| TEXAS INSTRUMENTS INCORPORATED
| Standard Linear and Logic Group
| IBIS Model of SN74CBTLV3861
| LOW-VOLTAGE 10-BIT FET BUS SWITCH
| This file contains package information for the following:
|  TSSOP 24-pin (PW) package as [Component] CBTLV3861_PW
|  TVSOP 24-pin (DGV) package as [Component] CBTLV3861_DGV
|  SOIC 24-pin (DW) package as [Component] CBTLV3861_DW
|  SOP 24-pin (NS) package as [Component] CBTLV3861_NS
|  SSOP 24-pin (DBQ) package as [Component] CBTLV3861_DBQ
| This device can be powered at the following Vccs:
|  3.3 volt Vcc
|  2.5 volt Vcc
| This file provides unique models under the [Model Selector] for each Vcc.
| For operation at a specific Vcc, select the appropriate model after each
| [Model Selector] keyword.
[IBIS Ver]   3.2
[Comment char]  |_char
[File Name]   sn74cbtlv3861.ibs
[File Rev]   1.0 | x_die
[Date]   May 11, 2009
[Source]   Data created from TI-SPICE simulations at TI-SLL.
[Notes]   The following is an IBIS list for the SN74CBTLV3861.
   Please contact sllibis@ti.com with questions and
   comments concerning SLL IBIS models.
   -FILE REV HISTORY
   -1.0 Release IBIS file on 05/11/09.
   -Power clamp data deleted as there is no power-clamp diode.
[Disclaimer] Property of Texas Instruments Incorporated.  Unauthorized
   reproduction and/or distribution is strictly prohibited.
   This product is protected under copyright law.
   Created  2007, (C) Copyright  2007, Texas Instruments
   Incorporated, All Rights Reserved
   UNLESS THERE IS A SIGNED, WRITTEN AGREEMENT TO THE
   CONTRARY, TEXAS INSTRUMENTS (TI) IS PROVIDING THE IBIS
   MODELS  AND WITHOUT ANY WARRANTY, EXPRESSED OR
   IMPLIED.  TI assumes no liability for:
   1) the accuracy of the IBIS models provided to your
   company;
   2) the proper functioning of these IBIS Models in your
   design or for any resulting applications; or
   3) infringement of patents, copyrights or intellectual
   property rights resulting from your use of these IBIS
   models.
   TI provides IBIS Models as a service to our customers.
   You and your company shall not distribute, sell or give
   these models to anyone else without prior written
   permission from TI.
   TI reserves the right to make changes to our products or
   to discontinue any semiconductor product or service
   without notice, and advises our customers to obtain the
   latest version of relevant information to verify, before
   placing orders, that the information being relied on is
   current.
   Please be aware that your receipt and use of the IBIS
   information provided shall serve as acceptance of these
   terms and conditions.  If you do not accept these terms,
   you should return or destroy the IBIS models and any
   other accompanying information immediately.
| Component SN74CBTLV3861_PW 24-PIN TSSOP
[Component]   SN74CBTLV3861_PW
[Manufacturer]   Texas Instruments, Inc.
[Package]
|   typ   min   max
R_pkg   3.900e-02   3.000e-02   4.600e-02
L_pkg   2.685e-09   2.367e-09   3.177e-09
C_pkg   3.200e-13   2.520e-13   4.340e-13
[Pin]   signal_name   model_name   R_pin   L_pin   C_pin
1   NC   NC   3.700e-02   3.153e-09   4.340e-13
2   A1   CBTLV3861_IO   3.400e-02   2.629e-09   3.410e-13
3   A2   CBTLV3861_IO   3.200e-02   2.860e-09   3.470e-13
4   A3   CBTLV3861_IO   4.200e-02   2.741e-09   2.900e-13
5   A4   CBTLV3861_IO   4.600e-02   2.600e-09   2.620e-13
6   A5   CBTLV3861_IO   4.300e-02   2.414e-09   2.660e-13
7   A6   CBTLV3861_IO   4.200e-02   2.367e-09   2.620e-13
8   A7   CBTLV3861_IO   4.400e-02   2.461e-09   2.520e-13
9   A8   CBTLV3861_IO   4.200e-02   2.543e-09   2.740e-13
10   A9   CBTLV3861_IO   3.000e-02   2.616e-09   3.320e-13
11   A10   CBTLV3861_IO   3.700e-02   2.670e-09   3.460e-13
12   GND   GND   3.900e-02   3.177e-09   4.330e-13
13   B10   CBTLV3861_IO   3.700e-02   3.111e-09   4.310e-13
14   B9   CBTLV3861_IO   3.700e-02   2.656e-09   3.450e-13
15   B8   CBTLV3861_IO   3.100e-02   2.739e-09   3.400e-13
16   B7   CBTLV3861_IO   4.200e-02   2.649e-09   2.820e-13
17   B6   CBTLV3861_IO   4.600e-02   2.532e-09   2.570e-13
18   B5   CBTLV3861_IO   4.400e-02   2.425e-09   2.660e-13
19   B4   CBTLV3861_IO   4.400e-02   2.425e-09   2.660e-13
20   B3   CBTLV3861_IO   4.600e-02   2.532e-09   2.570e-13
21   B2   CBTLV3861_IO   4.200e-02   2.648e-09   2.820e-13
22   B1   CBTLV3861_IO   3.100e-02   2.738e-09   3.390e-13
23   OE   CBTLV3861_IN   3.600e-02   2.653e-09   3.440e-13
24   VCC   POWER   3.700e-02   3.110e-09   4.310e-13
| Component SN74CBTLV3861_DGV 24-PIN TVSOP
[Component]   SN74CBTLV3861_DGV
[Manufacturer]   Texas Instruments, Inc.
[Package]
|   typ   min   max
R_pkg   4.300e-02   3.900e-02   4.700e-02
L_pkg   2.601e-09   2.312e-09   3.626e-09
C_pkg   3.580e-13   2.770e-13   5.950e-13
[Pin]   signal_name   model_name   R_pin   L_pin   C_pin
1   NC   NC   4.300e-02   3.625e-09   5.950e-13
2   A1   CBTLV3861_IO   4.000e-02   2.656e-09   4.020e-13
3   A2   CBTLV3861_IO   3.900e-02   2.338e-09   3.080e-13
4   A3   CBTLV3861_IO   4.600e-02   2.354e-09   2.770e-13
5   A4   CBTLV3861_IO   4.500e-02   2.312e-09   2.850e-13
6   A5   CBTLV3861_IO   4.700e-02   2.318e-09   2.820e-13
7   A6   CBTLV3861_IO   4.700e-02   2.318e-09   2.820e-13
8   A7   CBTLV3861_IO   4.500e-02   2.312e-09   2.850e-13
9   A8   CBTLV3861_IO   4.600e-02   2.353e-09   2.780e-13
10   A9   CBTLV3861_IO   3.900e-02   2.338e-09   3.080e-13
11   A10   CBTLV3861_IO   4.100e-02   2.660e-09   4.020e-13
12   GND   GND   4.300e-02   3.625e-09   5.950e-13
13   B10   CBTLV3861_IO   4.400e-02   3.626e-09   5.940e-13
14   B9   CBTLV3861_IO   4.000e-02   2.658e-09   4.020e-13
15   B8   CBTLV3861_IO   3.900e-02   2.343e-09   3.110e-13
16   B7   CBTLV3861_IO   4.600e-02   2.353e-09   2.780e-13
17   B6   CBTLV3861_IO   4.500e-02   2.312e-09   2.850e-13
18   B5   CBTLV3861_IO   4.700e-02   2.319e-09   2.820e-13
19   B4   CBTLV3861_IO   4.700e-02   2.319e-09   2.820e-13
20   B3   CBTLV3861_IO   4.500e-02   2.312e-09   2.850e-13
21   B2   CBTLV3861_IO   4.600e-02   2.353e-09   2.780e-13
22   B1   CBTLV3861_IO   3.900e-02   2.337e-09   3.080e-13
23   OE   CBTLV3861_IN   4.000e-02   2.658e-09   4.020e-13
24   VCC   POWER   4.400e-02   3.626e-09   5.950e-13
| Component SN74CBTLV3861_DW 24-PIN SOIC
[Component]   SN74CBTLV3861_DW
[Manufacturer]   Texas Instruments, Inc.
[Package]
|   typ   min   max
R_pkg   3.700e-02   3.000e-02   4.700e-02
L_pkg   5.146e-09   3.993e-09   6.885e-09
C_pkg   7.580e-13   5.120e-13   1.067e-12
[Pin]   signal_name   model_name   R_pin   L_pin   C_pin
1   NC   NC   3.900e-02   6.885e-09   1.067e-12
2   A1   CBTLV3861_IO   4.200e-02   5.950e-09   9.580e-13
3   A2   CBTLV3861_IO   4.700e-02   5.317e-09   7.910e-13
4   A3   CBTLV3861_IO   3.100e-02   4.651e-09   6.110e-13
5   A4   CBTLV3861_IO   3.000e-02   3.993e-09   5.120e-13
6   A5   CBTLV3861_IO   3.000e-02   4.083e-09   6.110e-13
7   A6   CBTLV3861_IO   3.000e-02   4.083e-09   6.110e-13
8   A7   CBTLV3861_IO   3.000e-02   3.993e-09   5.120e-13
9   A8   CBTLV3861_IO   3.100e-02   4.652e-09   6.110e-13
10   A9   CBTLV3861_IO   4.700e-02   5.317e-09   7.910e-13
11   A10   CBTLV3861_IO   4.200e-02   5.950e-09   9.590e-13
12   GND   GND   3.900e-02   6.885e-09   1.067e-12
13   B10   CBTLV3861_IO   3.900e-02   6.885e-09   1.067e-12
14   B9   CBTLV3861_IO   4.200e-02   5.950e-09   9.590e-13
15   B8   CBTLV3861_IO   4.700e-02   5.317e-09   7.910e-13
16   B7   CBTLV3861_IO   3.100e-02   4.652e-09   6.110e-13
17   B6   CBTLV3861_IO   3.000e-02   3.993e-09   5.120e-13
18   B5   CBTLV3861_IO   3.000e-02   4.083e-09   6.100e-13
19   B4   CBTLV3861_IO   3.000e-02   4.083e-09   6.100e-13
20   B3   CBTLV3861_IO   3.000e-02   3.993e-09   5.120e-13
21   B2   CBTLV3861_IO   3.100e-02   4.651e-09   6.110e-13
22   B1   CBTLV3861_IO   4.700e-02   5.317e-09   7.910e-13
23   OE   CBTLV3861_IN   4.200e-02   5.950e-09   9.580e-13
24   VCC   POWER   3.900e-02   6.885e-09   1.067e-12
| Component SN74CBTLV3861_NS 24-PIN SOP
[Component]   SN74CBTLV3861_NS
[Manufacturer]   Texas Instruments, Inc.
[Package]
|   typ   min   max
R_pkg   4.400e-02   3.800e-02   4.800e-02
L_pkg   3.840e-09   2.545e-09   5.234e-09
C_pkg   5.860e-13   2.740e-13   7.970e-13
[Pin]   signal_name   model_name   R_pin   L_pin   C_pin
1   NC   NC   4.100e-02   5.146e-09   7.650e-13
2   A1   CBTLV3861_IO   4.100e-02   4.357e-09   7.490e-13
3   A2   CBTLV3861_IO   4.000e-02   3.923e-09   6.330e-13
4   A3   CBTLV3861_IO   4.400e-02   3.412e-09   5.370e-13
5   A4   CBTLV3861_IO   4.500e-02   3.036e-09   3.970e-13
6   A5   CBTLV3861_IO   4.500e-02   2.845e-09   4.150e-13
7   A6   CBTLV3861_IO   4.400e-02   2.843e-09   4.150e-13
8   A7   CBTLV3861_IO   4.500e-02   3.065e-09   3.990e-13
9   A8   CBTLV3861_IO   4.500e-02   3.529e-09   5.440e-13
10   A9   CBTLV3861_IO   4.100e-02   4.013e-09   6.390e-13
11   A10   CBTLV3861_IO   4.100e-02   4.358e-09   7.460e-13
12   GND   GND   4.400e-02   5.234e-09   7.670e-13
13   B10   CBTLV3861_IO   3.900e-02   5.181e-09   7.650e-13
14   B9   CBTLV3861_IO   4.800e-02   4.582e-09   7.640e-13
15   B8   CBTLV3861_IO   4.100e-02   4.163e-09   6.550e-13
16   B7   CBTLV3861_IO   4.600e-02   3.613e-09   5.490e-13
17   B6   CBTLV3861_IO   4.700e-02   3.163e-09   4.060e-13
18   B5   CBTLV3861_IO   4.700e-02   2.963e-09   4.220e-13
19   B4   CBTLV3861_IO   4.700e-02   2.919e-09   4.190e-13
20   B3   CBTLV3861_IO   4.800e-02   3.087e-09   4.870e-13
21   B2   CBTLV3861_IO   4.600e-02   4.513e-09   7.600e-13
22   B1   CBTLV3861_IO   4.200e-02   4.505e-09   7.670e-13
23   OE   CBTLV3861_IN   4.200e-02   5.163e-09   7.970e-13
24   VCC   POWER   3.800e-02   2.545e-09   2.740e-13
| Component SN74CBTLV3861_DBQ 24-PIN SSOP
[Component]   SN74CBTLV3861_DBQ
[Manufacturer]   Texas Instruments, Inc.
[Package]
|   typ   min   max
R_pkg   4.400e-02   3.100e-02   6.600e-02
L_pkg   3.074e-09   2.348e-09   4.044e-09
C_pkg   3.220e-13   2.340e-13   4.460e-13
[Pin]   signal_name   model_name   R_pin   L_pin   C_pin
1   NC   NC   6.500e-02   4.044e-09   4.290e-13
2   A1   CBTLV3861_IO   6.600e-02   3.824e-09   4.460e-13
3   A2   CBTLV3861_IO   3.100e-02   3.011e-09   3.210e-13
4   A3   CBTLV3861_IO   3.200e-02   2.699e-09   2.590e-13
5   A4   CBTLV3861_IO   3.500e-02   2.519e-09   2.450e-13
6   A5   CBTLV3861_IO   3.500e-02   2.348e-09   2.340e-13
7   A6   CBTLV3861_IO   3.500e-02   2.348e-09   2.340e-13
8   A7   CBTLV3861_IO   3.500e-02   2.518e-09   2.450e-13
9   A8   CBTLV3861_IO   3.200e-02   2.699e-09   2.590e-13
10   A9   CBTLV3861_IO   3.100e-02   3.011e-09   3.210e-13
11   A10   CBTLV3861_IO   6.600e-02   3.824e-09   4.460e-13
12   GND   GND   6.500e-02   4.044e-09   4.290e-13
13   B10   CBTLV3861_IO   6.500e-02   4.044e-09   4.290e-13
14   B9   CBTLV3861_IO   6.600e-02   3.824e-09   4.460e-13
15   B8   CBTLV3861_IO   3.100e-02   3.011e-09   3.210e-13
16   B7   CBTLV3861_IO   3.200e-02   2.699e-09   2.590e-13
17   B6   CBTLV3861_IO   3.500e-02   2.518e-09   2.450e-13
18   B5   CBTLV3861_IO   3.500e-02   2.348e-09   2.340e-13
19   B4   CBTLV3861_IO   3.500e-02   2.348e-09   2.340e-13
20   B3   CBTLV3861_IO   3.500e-02   2.518e-09   2.450e-13
21   B2   CBTLV3861_IO   3.200e-02   2.699e-09   2.590e-13
22   B1   CBTLV3861_IO   3.100e-02   3.011e-09   3.210e-13
23   OE   CBTLV3861_IN   6.600e-02   3.824e-09   4.460e-13
24   VCC   POWER   6.500e-02   4.044e-09   4.290e-13
[Series Switch Groups]
| Function Group States
On  1 /   | A1-A10->B1-B10 NOE LOW
On  1 /   | NOE LOW
[Series Pin Mapping]   pin_2   model_name   function_table_group
2   22   CBTLV3861_IO_33_S   1
| 2   22   CBTLV3861_IO_25_S   1
3   21   CBTLV3861_IO_33_S   1
| 3   21   CBTLV3861_IO_25_S   1
4   20   CBTLV3861_IO_33_S   1
| 4   20   CBTLV3861_IO_25_S   1
5   19   CBTLV3861_IO_33_S   1
| 5   19   CBTLV3861_IO_25_S   1
6   18   CBTLV3861_IO_33_S   1
| 6   18   CBTLV3861_IO_25_S   1
7   17   CBTLV3861_IO_33_S   1
| 7   17   CBTLV3861_IO_25_S   1
8   16   CBTLV3861_IO_33_S   1
| 8   16   CBTLV3861_IO_25_S   1
9   15   CBTLV3861_IO_33_S   1
| 9   15   CBTLV3861_IO_25_S   1
10   14   CBTLV3861_IO_33_S   1
| 10   14   CBTLV3861_IO_25_S   1
11   13   CBTLV3861_IO_33_S   1
| 11   13   CBTLV3861_IO_25_S   1
| Model CBTLV3861_IN
[Model Selector]   CBTLV3861_IN
CBTLV3861_IN_33   3.3 volt Vcc
CBTLV3861_IN_25   2.5 volt Vcc
| Model CBTLV3861_IO
[Model Selector]   CBTLV3861_IO
CBTLV3861_IO_33   3.3 volt Vcc
CBTLV3861_IO_25   2.5 volt Vcc
[Model]   CBTLV3861_IO_33_S
Model_type  Series_switch
| variable   typ   min   max
C_comp   0   0   0
[Temperature Range]   40   100   -40
| Ambient temperature   25   85   -40
[Voltage range]   3.3   3   3.6
[On]
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[Off]
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[Model]   CBTLV3861_IO_25_S
Model_type  Series_switch
| variable   typ   min   max
C_comp   0   0   0
[Temperature Range]   40   100   -40
| Ambient temperature   25   85   -40
[Voltage range]   2.5   2.3   2.7
[On]
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[Off]
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| Models and submodels in the file (6): CBTLV3861_IN_33 (Input), CBTLV3861_IN_25 (Input), CBTLV3861_IO_33_S (Series_switch), CBTLV3861_IO_33 (Terminator), CBTLV3861_IO_25_S (Series_switch), CBTLV3861_IO_25 (Terminator)
